DATA_BLOCK "DatiVari"
VERSION : 0.1


  STRUCT
   TempoLavoroApeMandrino : S5TIME ;	//Tempo lavoro richiamo apertura mandrino
   TempoPausaApeMandrino : S5TIME ;	//Tempo pausa richiamo apertura mandrino
   SpessoreLama : DWORD ;	//Spessore lama
  END_STRUCT ;
BEGIN
   TempoLavoroApeMandrino := S5T#3S;
   TempoPausaApeMandrino := S5T#5M;
   SpessoreLama := DW#16#0;
END_DATA_BLOCK

